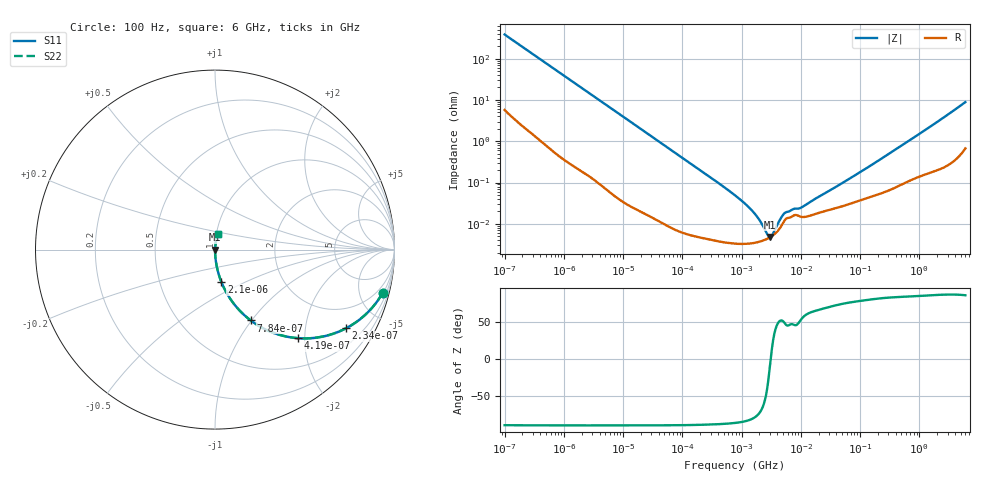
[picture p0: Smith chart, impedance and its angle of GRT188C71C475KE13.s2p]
!Murata Part Number: GRT188C71C475KE13
!These Parameters are Measured in Series Mode Connection
!Data Generated on Jun 19, 2026
!  o--ll--o
!Port1  Port2
!  o------o
!Operation Temp=25[degC], DC Bias Voltage=0[V]
!Freq. Start=100[Hz] Stop=6[GHz] 401[Steps]
# Hz S RI R 50
!Freq.(Hz) S11(Real) S11(Imag) S21(Real) S21(Imag) S12(Real) S12(Imag) S22(Real) S22(Imag)
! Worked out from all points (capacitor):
!   401 points, 100 Hz to 6 GHz, reference 50 ohm
!   read as one part in series: C = 4.14 uF near 109 Hz
!   lowest |Z| = 4.81 mohm at 2.968 MHz (marker M1)
!   S11 on the Smith chart (normalised r, x): 100 Hz: 1.11, -7.68; 234 Hz: 1.04, -3.30; 419 Hz: 1.02, -1.85; 784 Hz: 1.01, -0.99; 2.1 kHz: 1.00, -0.37; 6 GHz: 1.01, +0.18
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100  0.9333 -0.2421  0.0667 0.2421  0.0667 0.2421  0.9333 -0.2421
150  0.8656 -0.3348  0.1344 0.3348  0.1344 0.3348  0.8656 -0.3348
234  0.7286 -0.4388  0.2714 0.4388  0.2714 0.4388  0.7286 -0.4388
419  0.4613 -0.4933  0.5387 0.4933  0.5387 0.4933  0.4613 -0.4933
784  0.1995 -0.395  0.8005 0.395  0.8005 0.395  0.1995 -0.395
1227  0.0937 -0.2869  0.9063 0.2869  0.9063 0.2869  0.0937 -0.2869
2008  0.0381 -0.1868  0.9619 0.1868  0.9619 0.1868  0.0381 -0.1868
2100  0.0351 -0.1792  0.9649 0.1792  0.9649 0.1792  0.0351 -0.1792
6728  0.00391 -0.0582  0.9961 0.0582  0.9961 0.0582  0.00391 -0.0582
40335  0.000212 -0.00984  0.9998 0.00984  0.9998 0.00984  0.000212 -0.00984
774597  3.34e-05 -0.00049  1 0.00049  1 0.00049  3.34e-05 -0.00049
1386327  3.35e-05 -0.000234  1 0.000234  1 0.000234  3.35e-05 -0.000234
2169299  3.82e-05 -9.6e-05  1 9.6e-05  1 9.6e-05  3.82e-05 -9.6e-05
2372521  4e-05 -7.14e-05  1 7.14e-05  1 7.14e-05  4e-05 -7.14e-05
2967816  4.66e-05 -1.18e-05  1 1.18e-05  1 1.18e-05  4.66e-05 -1.18e-05
3882480  6.25e-05 6.04e-05  0.9999 -6.04e-05  0.9999 -6.04e-05  6.25e-05 6.04e-05
5554849  0.000131 0.000138  0.9999 -0.000138  0.9999 -0.000138  0.000131 0.000138
9941735  0.000149 0.000192  0.9999 -0.000192  0.9999 -0.000192  0.000149 0.000192
1.555665e7  0.000164 0.000326  0.9998 -0.000326  0.9998 -0.000326  0.000164 0.000326
3.124326e8  0.000676 0.005  0.9993 -0.005  0.9993 -0.005  0.000676 0.005
1.873145e9  0.00264 0.0272  0.9974 -0.0272  0.9974 -0.0272  0.00264 0.0272
6e9  0.0143 0.0865  0.9857 -0.0865  0.9857 -0.0865  0.0143 0.0865
